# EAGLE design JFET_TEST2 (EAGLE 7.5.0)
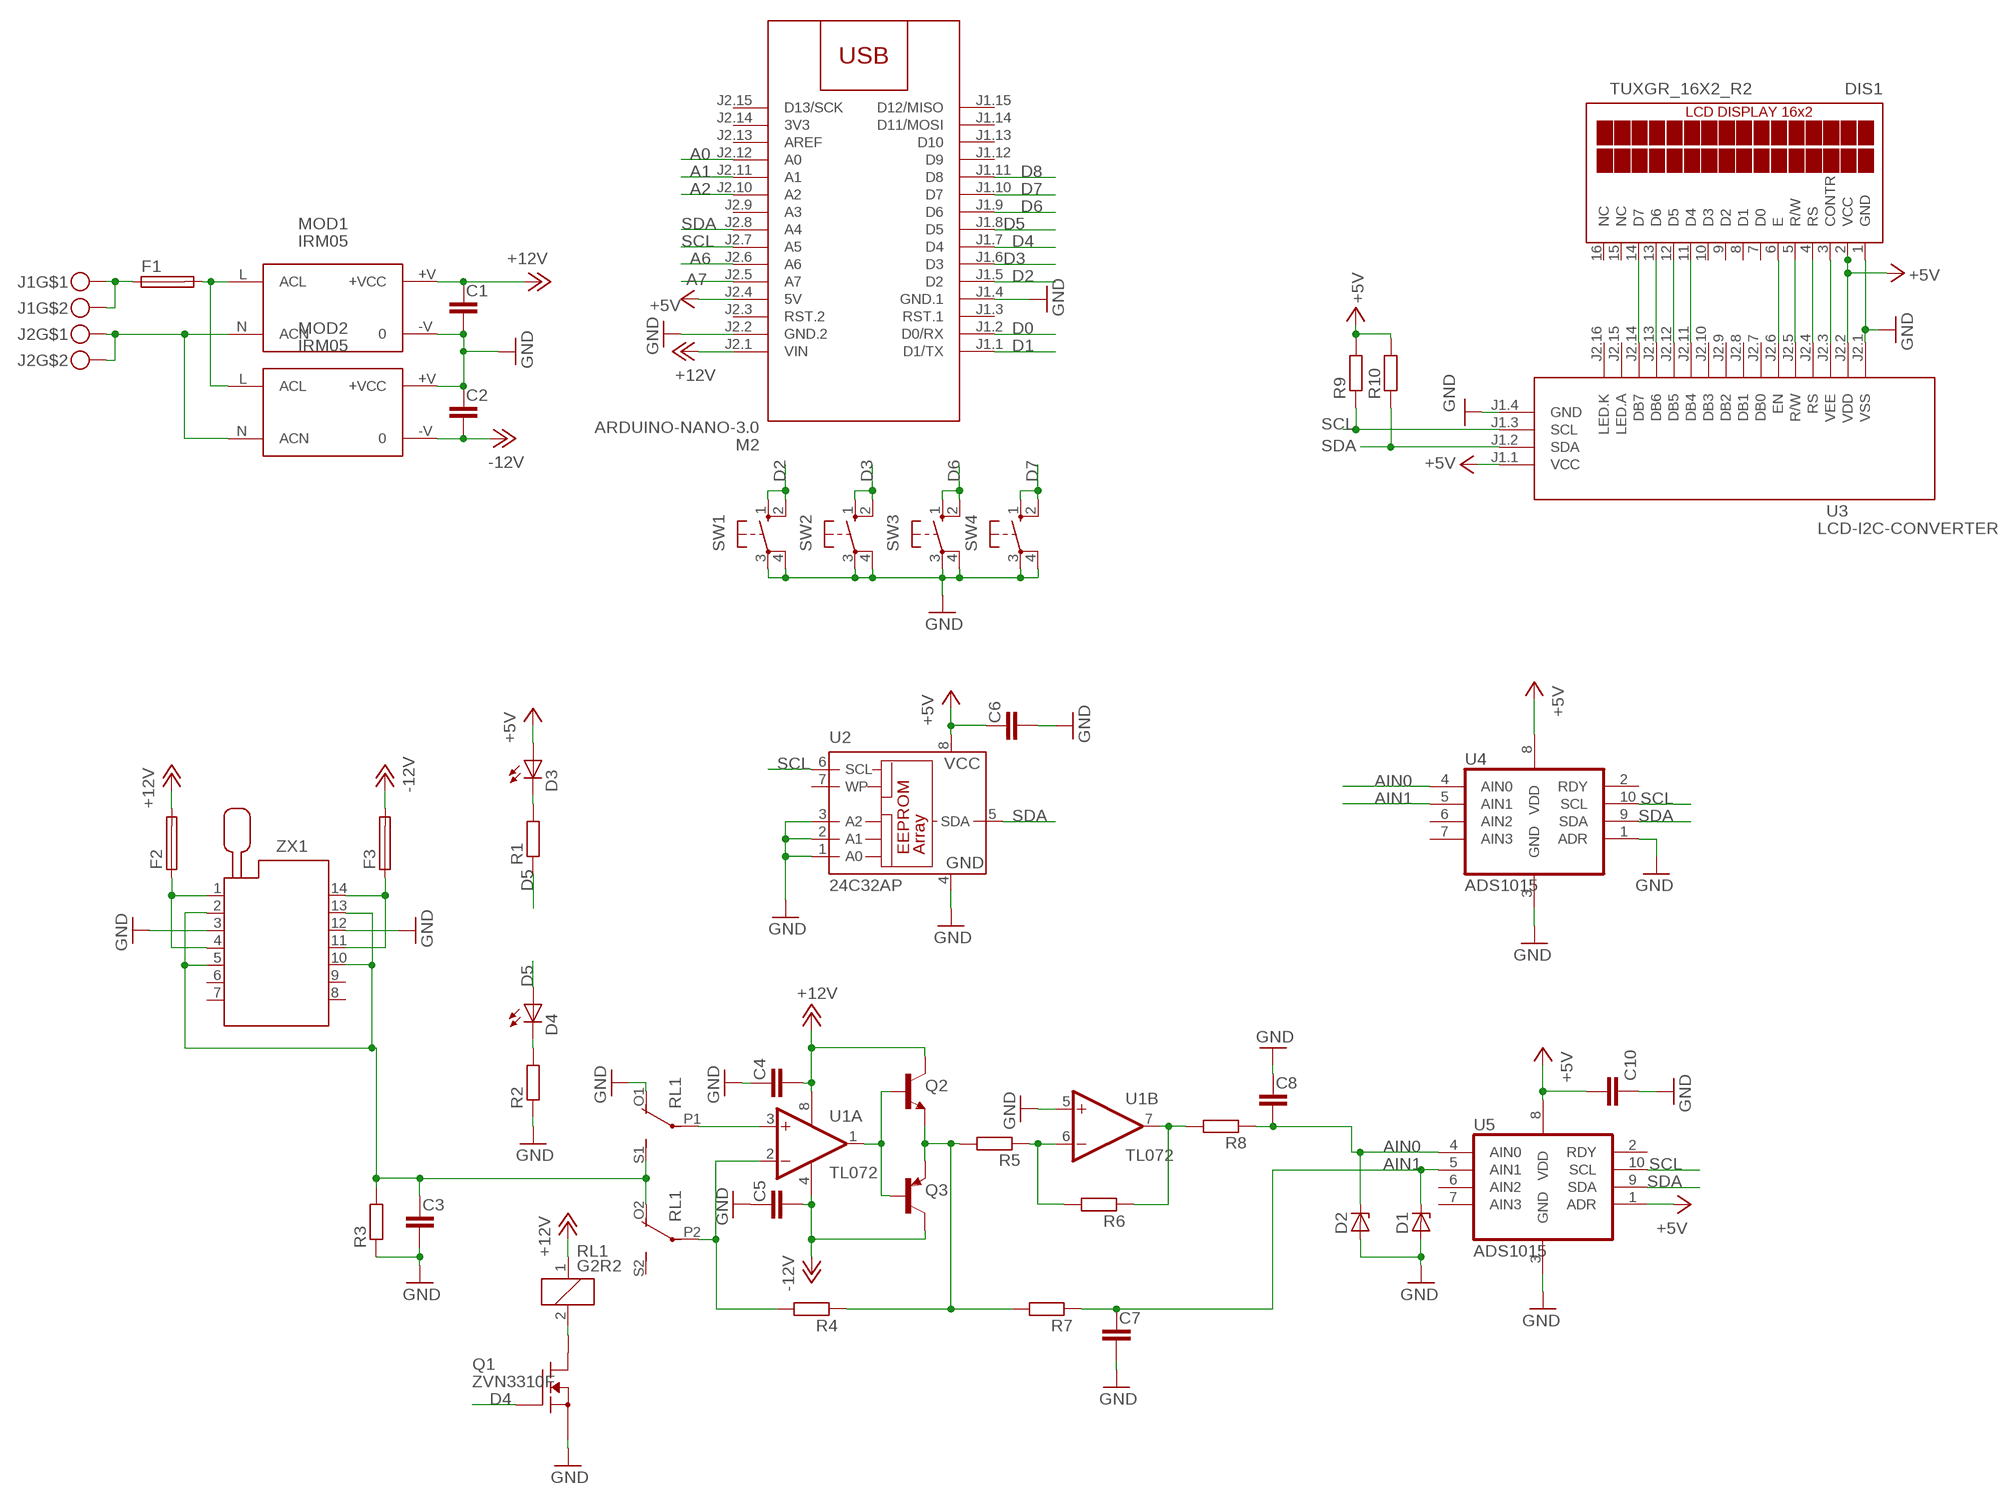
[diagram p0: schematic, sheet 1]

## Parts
C1  C-EUC1206  [C1206]
C2  C-EUC1206  [C1206]
C3  C-EUC1206  [C1206]
C4  C-EUC1206  [C1206]
C5  C-EUC1206  [C1206]
C6  C-EUC1206  [C1206]
C7  C-EUC1206  [C1206]
C8  C-EUC1206  [C1206]
C10  C-EUC1206  [C1206]
D1  BZX84CSMD  [TO236]
D2  BZX84CSMD  [TO236]
D3  LED5MM  [LED5MM]
D4  LED5MM  [LED5MM]
DIS1  TUXGR_16X2_R2  [TUXGR_16X2_R2]
F1  FUSEBLANK_5X20MM  [FUSE_HOLDER_5X20MM]
F2  FUSEBLANK_5X20MM  [FUSE_HOLDER_5X20MM]
F3  FUSEBLANK_5X20MM  [FUSE_HOLDER_5X20MM]
J1  MKDSN1,5-2-5,08  [MKDSN1,5-2-5,08]
J2  MKDSN1,5-2-5,08  [MKDSN1,5-2-5,08]
M2  ARDUINO-NANO-3.0  [ARDUINO-NANO-3.0]
MOD1  IRM05  [IRM05]
MOD2  IRM05  [IRM05]
Q1  ZVN3310F  BSS138  [SOT23]
Q2  BC817-40LT1SMD  [SOT23-BEC]
Q3  BC858ALT1SMD  [SOT23-BEC]
R1  R-EU_R1206  [R1206]
R2  R-EU_R1206  [R1206]
R3  R-EU_R1206  [R1206]
R4  R-EU_R1206  [R1206]
R5  R-EU_R1206  [R1206]
R6  R-EU_R1206  [R1206]
R7  R-EU_R1206  [R1206]
R8  R-EU_R1206  [R1206]
R9  R-EU_R1206  [R1206]
R10  R-EU_R1206  [R1206]
RL1  G2R2  [G2R2]
SW1  40-XX  [B3F-40XX]
SW2  40-XX  [B3F-40XX]
SW3  40-XX  [B3F-40XX]
SW4  40-XX  [B3F-40XX]
U1  TL072  OPA2134PA  [DIL08]
U2  24C32AP  [DIL8]
U3  LCD-I2C-CONVERTER  [LCD-I2C-CONVERTER]
U4  ADS1015  [ADS1015]
U5  ADS1015  [ADS1015]
ZX1  214-3339-00-0602J  [214-3339-00-0602J]

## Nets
+5V: C6.1 C10.2 D3.A DIS1.2(VCC) M2.J2.4(5V) R9.2 R10.2 U2.8(VCC) U3.J1.1(VCC) U3.J2.2(VDD) U4.8(VDD) U5.1(ADR) U5.8(VDD)
+12V: C1.1 C4.2 F2.2 M2.J2.1(VIN) MOD1.+V(+VCC) Q2.C RL1.1 U1.8(A:V+)
-12V: C2.2 C5.2 F3.2 MOD2.-V Q3.C U1.4(A:V-)
A0: M2.J2.12(A0)
A1: M2.J2.11(A1)
A2: M2.J2.10(A2)
A6: M2.J2.6(A6)
A7: M2.J2.5(A7)
AIN0: C8.2 D2.C R8.1 U4.4(AIN0) U5.4(AIN0)
AIN1: C7.1 D1.C R7.1 U4.5(AIN1) U5.5(AIN1)
D0: M2.J1.2(D0/RX)
D1: M2.J1.1(D1/TX)
D2: M2.J1.5(D2) SW1.1(S) SW1.2(S1)
D3: M2.J1.6(D3) SW2.1(S) SW2.2(S1)
D4: M2.J1.7(D4) Q1.3(G)
D5: D4.A M2.J1.8(D5) R1.1
D6: M2.J1.9(D6) SW3.1(S) SW3.2(S1)
D7: M2.J1.10(D7) SW4.1(S) SW4.2(S1)
D8: M2.J1.11(D8)
GND: C1.2 C2.1 C3.2 C4.1 C5.1 C6.2 C7.2 C8.1 C10.1 D1.A D2.A DIS1.1(GND) M2.J1.4(GND.1) M2.J2.2(GND.2) MOD1.-V MOD2.+V(+VCC) Q1.1(S) R2.1 R3.1 RL1.O1(2:O) SW1.3(P) SW1.4(P1) SW2.3(P) SW2.4(P1) SW3.3(P) SW3.4(P1) SW4.3(P) SW4.4(P1) U1.5(B:+IN) U2.1(A0) U2.2(A1) U2.3(A2) U2.4(GND) U3.J1.4(GND) U3.J2.1(VSS) U4.1(ADR) U4.3(GND) U5.3(GND) ZX1.3 ZX1.12
N$1: DIS1.14(D7) U3.J2.14(DB7)
N$2: DIS1.13(D6) U3.J2.13(DB6)
N$3: DIS1.12(D5) U3.J2.12(DB5)
N$4: DIS1.11(D4) U3.J2.11(DB4)
N$5: DIS1.6(E) U3.J2.6(EN)
N$6: DIS1.5(R/W) U3.J2.5(R/W)
N$7: DIS1.4(RS) U3.J2.4(RS)
N$10: DIS1.3(CONTR) U3.J2.3(VEE)
N$11: C3.1 R3.2 RL1.O2(3:O) RL1.S1(2:S) ZX1.2 ZX1.5 ZX1.10 ZX1.13
N$13: D4.K(C) R2.2
N$14: D3.K(C) R1.2
N$15: Q1.2(D) RL1.2
N$16: RL1.P1(2:P) U1.3(A:+IN)
N$17: R4.2 RL1.P2(3:P) U1.2(A:-IN)
N$18: Q2.B Q3.B U1.1(A:OUT)
N$19: Q2.E Q3.E R4.1 R5.2 R7.2
N$20: F1.1 J1.1 J1.2
N$21: F1.2 MOD1.L(ACL) MOD2.L(ACL)
N$24: R5.1 R6.2 U1.6(B:-IN)
N$25: R6.1 R8.2 U1.7(B:OUT)
N$26: J2.1 J2.2 MOD1.N(ACN) MOD2.N(ACN)
N$27: F2.1 ZX1.1 ZX1.4
N$28: F3.1 ZX1.11 ZX1.14
SCL: M2.J2.7(A5) R9.1 U2.6(SCL) U3.J1.3(SCL) U4.10(SCL) U5.10(SCL)
SDA: M2.J2.8(A4) R10.1 U2.5(SDA) U3.J1.2(SDA) U4.9(SDA) U5.9(SDA)
Unconnected: DIS1.7(D0) DIS1.8(D1) DIS1.9(D2) DIS1.10(D3) DIS1.15(NC) DIS1.16(NC) M2.J1.3(RST.1) M2.J1.12(D9) M2.J1.13(D10) M2.J1.14(D11/MOSI) M2.J1.15(D12/MISO) M2.J2.3(RST.2) M2.J2.9(A3) M2.J2.13(AREF) M2.J2.15(D13/SCK) RL1.S2(3:S) U2.7(WP) U3.J2.7(DB0) U3.J2.8(DB1) U3.J2.9(DB2) U3.J2.10(DB3) U3.J2.15(LED.A) U3.J2.16(LED.K) U4.2(RDY) U4.6(AIN2) U4.7(AIN3) U5.2(RDY) U5.6(AIN2) U5.7(AIN3) ZX1.6 ZX1.7 ZX1.8 ZX1.9

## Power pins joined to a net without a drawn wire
3V3: M2.J2.14(3V3)

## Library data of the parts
C1-C8 C10 = rcl:C-EU: CAPACITOR, European symbol
D1 D2 = diode:BZX84CSMD: Z DIODE
D3 D4 = led:LED: LED
DIS1 = display-lcd:TUXGR_16X2_R2: Tuxgraphics LCD display 16x2 characters reflective, without background light Source: tuxgr_12x2_r2.pdf; OC_FARNELL: unknown; OC_NEWARK: unknown
F1-F3 = fuse:FUSE: Fuse; OC_FARNELL: unknown; OC_NEWARK: unknown
J1 J2 = con-phoenix-508:MKDSN1,5-2-5,08
M2 = diy-modules:ARDUINO-NANO-3.0: Arduino Nano 3.0 and compatible devices More details available here: https://www.arduino.cc/en/Main/ArduinoBoardNano Click here to find device on ebay.com
MOD1 MOD2 = acdc:IRM05: ACDC connector
Q1 = transistor-fet:BSS138
Q2 = transistor-npn:BC817*: NPN Transistor
Q3 = transistor-pnp:BC858*: PNP Transistror
R1-R10 = rcl:R-EU_: RESISTOR, European symbol
RL1 = relay:G2R2: RELAY 2 x switch, Omron; MF: OMRON COMPONENTS USA; MPN: G2R-2-DC6; OC_FARNELL: unknown; OC_NEWARK: 89C5317
SW1-SW4 = switch-omron:40-XX: OMRON SWITCH; MF: OMRON COMPONENTS USA; MPN: B3F-4000; OC_FARNELL: 176434; OC_NEWARK: 36K3105
U1 = linear:OPA2*: Dual Operational Amplifier Low Power, Single-Supply, Rail-To-Rail Operational Amplifier Source: http://focus.ti.com/lit/ds/symlink/opa2345.pdf http://focus.ti.com .. opa241.pdf http://focus.ti.com/lit/ds/symlink/opa2134.pdf
U2 = microchip:24*: Serial EEPROM I2C; MPN: AT24C32C-PU; OC_FARNELL: 1362652; OC_NEWARK: 50M3325
U3 = diy-modules:LCD-I2C-CONVERTER: I2C Bus to 4-Bit Parallel LCD Interface with LED backlight driver
U4 U5 = burr-brown:ADS1015: 12BIT I2C DAC
ZX1 = con-3m:214-3339-00-0602J: Zero Insertion Force Socked Source: http://www.3M.com/ehpd; MF: 3M; MPN: 214-3339-00-0602J; OC_FARNELL: 1247151; OC_NEWARK: 85K7793

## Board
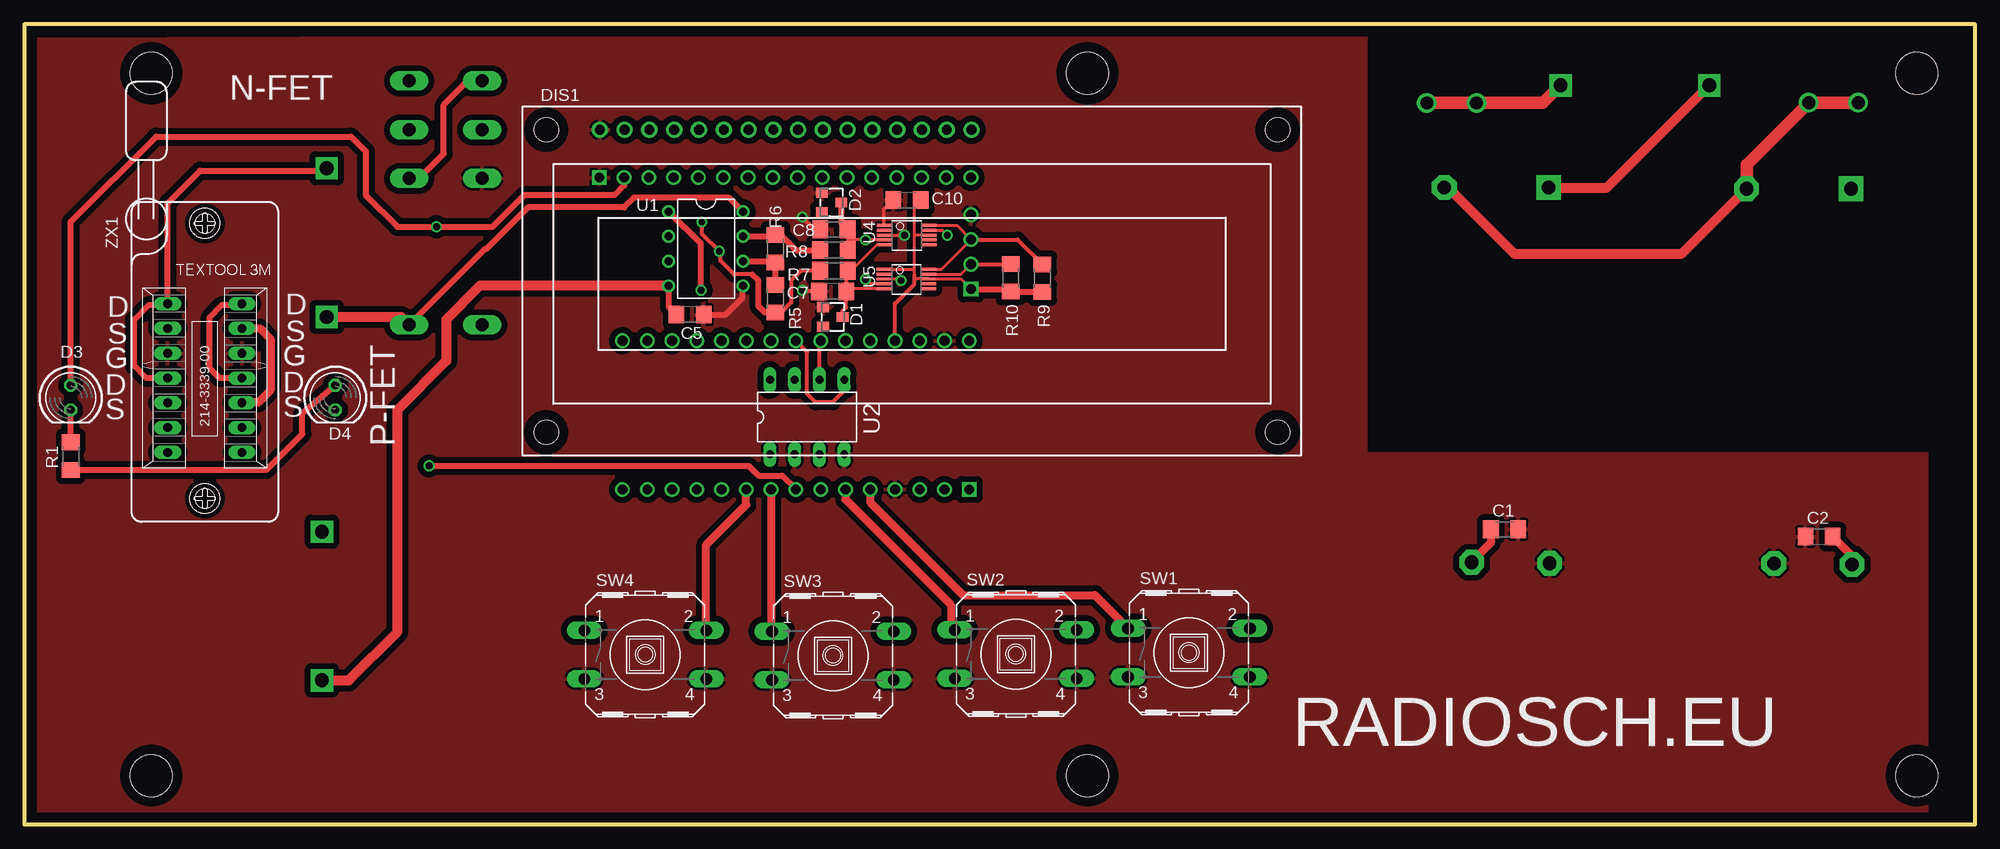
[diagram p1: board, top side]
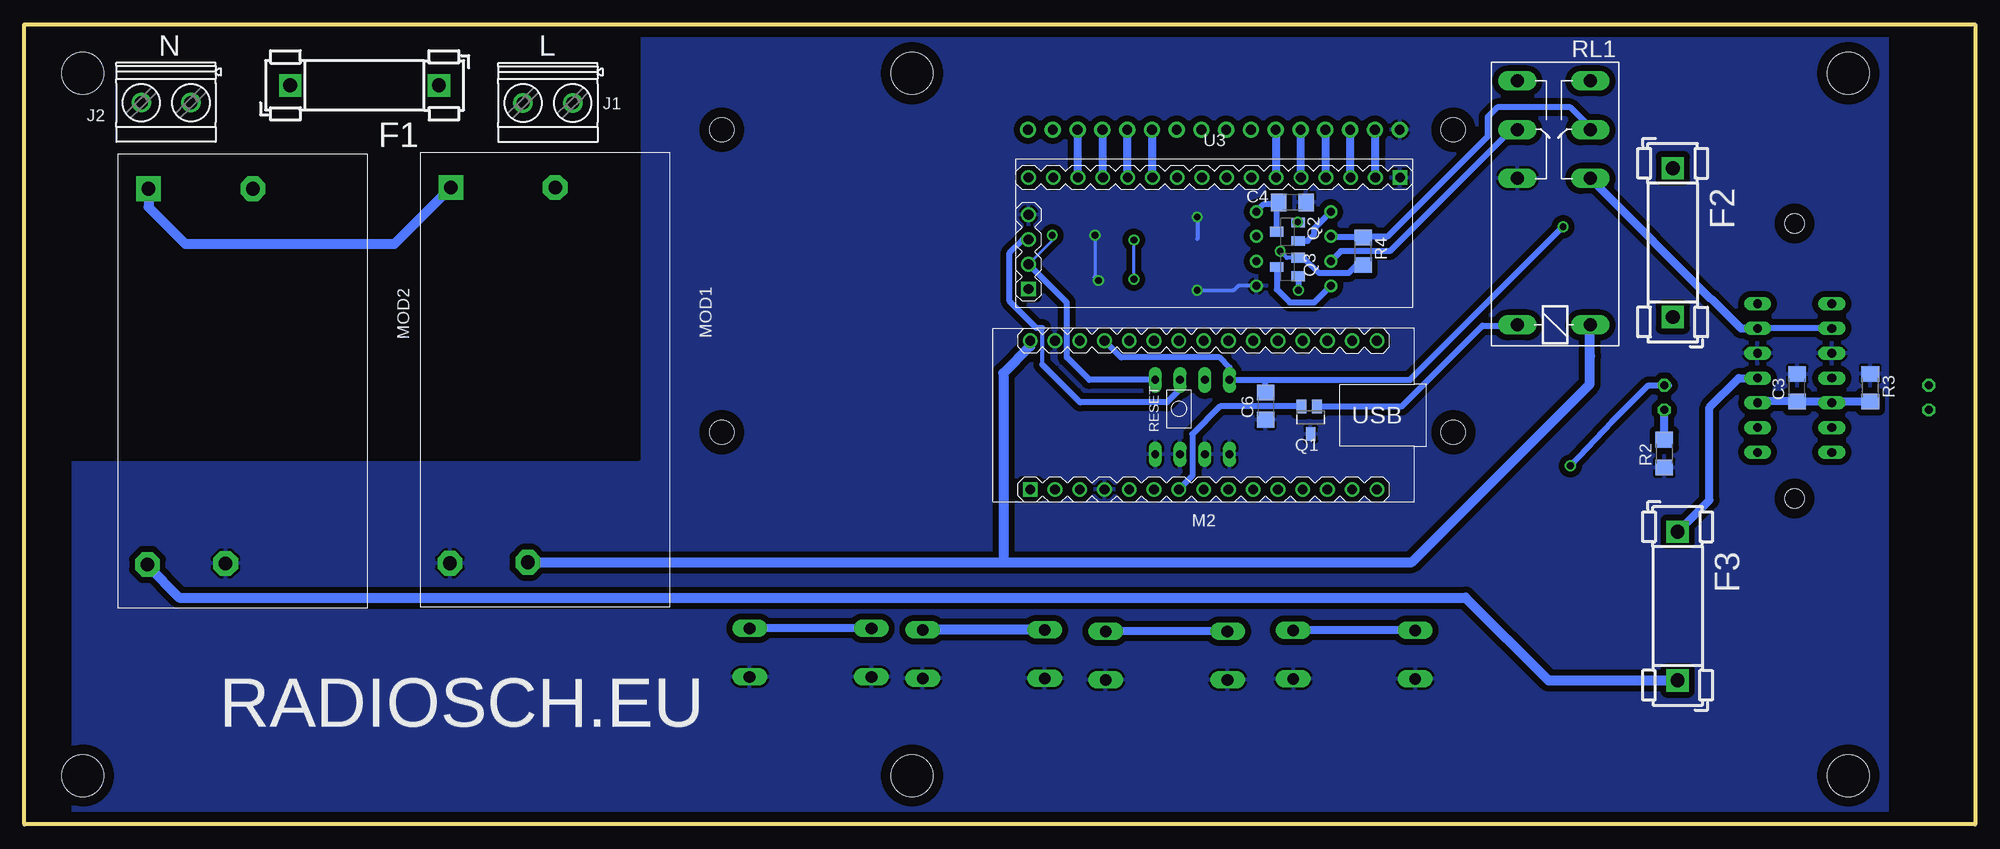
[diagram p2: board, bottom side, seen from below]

Size 200 x 82 mm. Coordinates in mm from the lower left corner, seen from the top.
Outline: 0,0 200,0 200,82 0,82 0,0
Copper layers (1*16): Top 0.035mm / dielectric 1.5mm / Bottom 0.035mm
Design rules "default *": minimum track width 10mil, minimum drill 24mil, track to track 4mil, track to pad 6mil, pad to pad 4mil, via to via 8mil, smd to smd 8mil, copper to edge 40mil, drill to drill 8mil, minimum pad ring 10mil, minimum via ring 8mil, stop-mask expansion 4mil, vias tented up to drill 0mil, thermal gap 10mil
Holes 4.3 mm at 13,77 13,5 109,5 194,5 109,77 194,77

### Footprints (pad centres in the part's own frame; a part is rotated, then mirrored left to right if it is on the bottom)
C1206 = smd 1.6 x 1.8: 1 -1.4,0; 2 1.4,0
TO236 = smd 1 x 1.2: A -1,-1; C 0,1; NC 1,-1
LED5MM = drill 0.813 octagon: A -1.27,0; K 1.27,0
TUXGR_16X2_R2 = drill 1 pad 1.676: 1 -32,15.5; 2 -29.46,15.5; 3 -26.92,15.5; 4 -24.38,15.5; 5 -21.84,15.5; 6 -19.3,15.5; 7 -16.76,15.5; 8 -14.22,15.5; 9 -11.68,15.5; 10 -9.14,15.5; 11 -6.6,15.5; 12 -4.06,15.5; 13 -1.52,15.5; 14 1.02,15.5; 15 3.56,15.5; 16 6.1,15.5 | hole 2.5: -37.5,-15.5; 37.5,-15.5; -37.5,15.5; 37.5,15.5
FUSE_HOLDER_5X20MM = drill 1.422 pad 2.286 square: 1 0,0; 2 15.24,0
MKDSN1,5-2-5,08 = drill 1.3 pad 2: 1 -2.561,0.025; 2 2.519,0.025
ARDUINO-NANO-3.0 = drill 1 square: J1.1 17.78,7.62 | drill 1: J1.2 15.24,7.62; J1.3 12.7,7.62; J1.4 10.16,7.62; J1.5 7.62,7.62; J1.6 5.08,7.62; J1.7 2.54,7.62; J1.8 0,7.62; J1.9 -2.54,7.62; J1.10 -5.08,7.62; J1.11 -7.62,7.62; J1.12 -10.16,7.62; J1.13 -12.7,7.62; J1.14 -15.24,7.62; J1.15 -17.78,7.62; J2.1 17.78,-7.62; J2.2 15.24,-7.62; J2.3 12.7,-7.62; J2.4 10.16,-7.62; J2.5 7.62,-7.62; J2.6 5.08,-7.62; J2.7 2.54,-7.62; J2.8 0,-7.62; J2.9 -2.54,-7.62; J2.10 -5.08,-7.62; J2.11 -7.62,-7.62; J2.12 -10.16,-7.62; J2.13 -12.7,-7.62; J2.14 -15.24,-7.62; J2.15 -17.78,-7.62
IRM05 = drill 1.4 pad 2.54 octagon: +V 42,-14.5; -V 42.1,-22.5; N 3.6,-11.7 | drill 1.4 pad 2.54 square: L 3.6,-22.4
SOT23 = smd 1 x 1.4: 1 0,1.735; 2 -0.632,-1.1; 3 0.95,-1.1
SOT23-BEC = smd 1 x 1.4: B -0.95,-1.1; C 0,1.1; E 0.95,-1.1
R1206 = smd 1.6 x 1.803: 1 -1.422,0; 2 1.422,0
G2R2 = drill 1.321 long: 1 -2.54,-3.683; 2 -2.54,3.81; O1 12.471,3.81; O2 12.471,-3.683; P1 17.45,3.81; P2 17.45,-3.683; S1 22.454,3.81; S2 22.454,-3.683
B3F-40XX = drill 1.194 long: 1 -6.248,2.489; 2 6.248,2.489; 3 -6.248,-2.489; 4 6.248,-2.489
DIL08 = drill 0.813 pad 1.27: 1 -3.81,-3.81; 2 -1.27,-3.81; 3 1.27,-3.81; 4 3.81,-3.81; 5 3.81,3.81; 6 1.27,3.81; 7 -1.27,3.81; 8 -3.81,3.81
DIL8 = drill 0.813 long: 1 -3.81,-3.81; 2 -1.27,-3.81; 3 1.27,-3.81; 4 3.81,-3.81; 5 3.81,3.81; 6 1.27,3.81; 7 -1.27,3.81; 8 -3.81,3.81
LCD-I2C-CONVERTER = drill 1 square: J1.1 -19.05,-5.08; J2.1 19.05,6.35 | drill 1: J1.2 -19.05,-2.54; J1.3 -19.05,0; J1.4 -19.05,2.54; J2.2 16.51,6.35; J2.3 13.97,6.35; J2.4 11.43,6.35; J2.5 8.89,6.35; J2.6 6.35,6.35; J2.7 3.81,6.35; J2.8 1.27,6.35; J2.9 -1.27,6.35; J2.10 -3.81,6.35; J2.11 -6.35,6.35; J2.12 -8.89,6.35; J2.13 -11.43,6.35; J2.14 -13.97,6.35; J2.15 -16.51,6.35; J2.16 -19.05,6.35
ADS1015 = smd 0.3 x 1.5: 1 -1.905,-2.616; 2 -1.405,-2.616; 3 -0.905,-2.616; 4 -0.405,-2.616; 5 0.095,-2.616; 6 0.095,1.984; 7 -0.405,1.984; 8 -0.905,1.984; 9 -1.405,1.984; 10 -1.905,1.984
214-3339-00-0602J = drill 0.9 long: 1 -7.62,-3.81; 2 -5.08,-3.81; 3 -2.54,-3.81; 4 0,-3.81; 5 2.54,-3.81; 6 5.08,-3.81; 7 7.62,-3.81; 8 7.62,3.81; 9 5.08,3.81; 10 2.54,3.81; 11 0,3.81; 12 -2.54,3.81; 13 -5.08,3.81; 14 -7.62,3.81 | hole 2: 12.35,0; -15.85,0

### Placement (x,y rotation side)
C1  151.75,30.25 0 top
C2  184,29.5 0 top
C3  18.25,44.75 90 bottom
C4  70,63.75 180 bottom
C5  68.25,52.25 180 top
C6  72.75,42.88 270 bottom
C7  82.88,54.62 180 top
C8  83,61 0 top
C10  90.5,64 0 top
D1  82.88,52 270 top
D2  82.75,63.75 270 top
D3  4.75,43.75 270 top
D4  31.88,43.75 270 top
DIS1  91,55.7 0 top
F1  157.5,75.75 180 bottom
F2  31,67.25 270 bottom
F3  30.5,30 270 bottom
J1  146.35,73.97 180 bottom
J2  185.5,74 180 bottom
M2  79.1,41.95 180 bottom
MOD1  133.88,68.88 270 bottom
MOD2  164.88,68.75 270 bottom
Q1  68.12,41.75 180 bottom
Q2  70.5,60.75 90 bottom
Q3  70.5,57.12 90 bottom
R1  4.75,37.75 90 top
R2  31.88,38 90 bottom
R3  10.75,44.75 270 bottom
R4  62.75,58.75 90 bottom
R5  77,53.88 270 top
R6  77,59 270 top
R7  83,56.75 180 top
R8  83,58.88 180 top
R9  104.38,55.97 270 top
R10  101.12,56.03 270 top
RL1  43.12,53.75 90 bottom
SW1  119.4,17.6 0 top
SW2  101.65,17.45 0 top
SW3  82.9,17.3 0 top
SW4  63.65,17.4 0 top
U1  69.88,59 270 top
U2  80.25,41.75 0 top
U3  78,59.95 0 bottom
U4  90.78,59.5 270 top
U5  90.75,55 270 top
ZX1  18.5,45.75 270 top

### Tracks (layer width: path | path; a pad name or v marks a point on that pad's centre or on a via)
+5V  (via drill 0.7)
  Top 0.305: U5.1 91.22,56.91 91.25,56.88 | 91.25,56.88 91.25,60.5 | 91.25,60.5 91.25,63.35 C10.2 | U4.8 91.34,60.41 91.25,60.5 | 91.25,56.88 91.25,56.25 91.25,56.12 91.47,55.91 U5.8 96.02,55.91 U3.J1.1
  Top 0.406: M2.J2.4 89.26,53.39 91.25,55.38 91.25,56.25
  Top 0.61: U3.J1.1 100.86,54.87 R10.2 104.33,54.6 R9.2 | U3.J2.2 61.49,65.49 60.5,64.5 51.25,64.5 48,61.25 v42.25,61.25 38.25,61.25 35,64.5 35,69 33.5,70.5 13.5,70.5 4.75,61.75 D3.A
  Bottom 0.61: M2.J2.4 87.56,47.88 77.5,47.88 76.44,46.81 U2.8 72.88,45.56 | 72.88,45.56 57.94,45.56 v42.25,61.25 | C6.1 72.75,45.44 72.88,45.56
  Bottom 0.813: U3.J2.2 61.49,71.15 DIS1.2
+12V
  Top 0.61: RL1.1 47.23,59 47.38,59 51.62,63.25 61.5,63.25 62.5,64.25 72.25,64.25 U1.8
  Top 0.813: C1.1 150.35,28.85 MOD1.+V
  Top 1.016: F2.2 38.64,52.01 RL1.1
  Bottom 0.61: Q2.C 71.6,63.55 | 71.6,63.55 C4.2 | 71.6,63.55 72.94,63.55 U1.8
  Bottom 1.016: MOD1.+V 99.62,26.88 | 99.62,26.88 57.75,26.88 39.5,45.12 39.5,48 | 39.5,48 39.5,51.15 RL1.1 | 39.49,48.01 39.5,48 | M2.J2.1 96.88,49 99.62,46.25 99.62,26.88
-12V
  Top 0.61: U1.4 66.06,53.03 C5.2
  Top 0.813: MOD2.-V 187.38,27.52 C2.2
  Top 1.016: U1.4 66,55.25 46.75,55.25 43.25,51.75 43.25,47.5 38.25,42.5 38.25,19.75 33.26,14.76 F3.2
  Bottom 0.61: Q3.C 71.6,54.85 70.25,53.5 67.75,53.5 U1.4
  Bottom 1.016: MOD2.-V 187.38,26.5 184.12,23.25 52.25,23.25 43.75,14.75 F3.2
AIN0  (via drill 0.7)
  Top 0.305: R8.1 84.42,59.75 | 84.42,59.75 84.42,60.98 C8.2 | U4.4 v86.25,59.91 84.58,59.91 84.42,59.75 | U5.4 86.72,55.41 v86.25,55.88
  Top 0.61: D2.C 83.75,61.65 C8.2
  Bottom 0.305: v86.25,55.88 v86.25,59.91
AIN1
  Top 0.305: U5.5 84.56,54.91 C7.1 | U4.5 87.41,59.41 85,57 84.67,57 R7.1
  Top 0.406: D1.C 83.88,52.62 84.25,53 84.25,54.6 C7.1 84.28,56.6 R7.1
D2
  Top 0.813: M2.J1.5 86.72,33.03 96.25,23.5 109.74,23.5 SW1.1
  Bottom 0.813: SW1.1 SW1.2
D3
  Top 0.813: M2.J1.6 84.18,33.32 95,22.5 95,20.34 SW2.1
  Bottom 1.016: SW2.1 SW2.2
D4
  Bottom 0.61: Q1.3 77.4,42.85 80.25,40 80.25,35.72 M2.J1.7
D5  (via drill 0.7)
  Top 0.61: v41.5,36.75 74.25,36.75 75.25,35.75 77.68,35.75 M2.J1.8 | D4.A 28.5,42.15 28.5,40 24.83,36.33 R1.1
  Bottom 0.61: v41.5,36.75 37.25,41.25 33.5,45 31.39,45 D4.A
D6
  Top 0.813: M2.J1.9 76.56,19.88 SW3.1
  Bottom 0.813: SW3.1 SW3.2
D7
  Top 0.813: SW4.2 69.9,28.65 74,32.75 74,34.31 M2.J1.10
  Bottom 0.813: SW4.1 SW4.2
GND  (via drill 0.7)
  Top 0.305: U5.3 90.03,55.91 v89.88,55.75 | U4.3 90.22,60.41 v90.25,60.38 | U4.1 88.16,62.09 88.12,62.12 88.12,63.12
  Top 0.406: 88.16,63.06 C10.1 | C7.2 79.88,54.62 v79.75,54.75 | C8.1 81,61 v79.75,62.25
  Top 0.61: C5.1 71.88,52.25 73.62,54 73.62,55.13 U1.5
  Bottom 0.305: 90.38,56.12 90,55.75 v89.88,55.75 90.25,56.12 v90.25,60.38
  Bottom 0.406: v79.75,54.75 76,54.75 75.5,55.25 73.75,55.25 U1.5 | v79.75,62.25 79.75,60
  pour Bottom (isolate 0.61): 9,81 195,81 195,1.5 9,1.5
  cutout Bottom: 137,81.5 195,81.5 195.5,37.5 137,37.5
  pour Top (isolate 0.61): 1,80.5 137.5,81 137.5,38 195,38 195,1 1,0.5
N$1
  Bottom 0.813: U3.J2.14 91.97,71.15 DIS1.14
N$2
  Bottom 0.813: U3.J2.13 89.43,71.15 DIS1.13
N$3
  Bottom 0.813: U3.J2.12 86.89,71.15 DIS1.12
N$4
  Bottom 0.813: U3.J2.11 84.35,71.15 DIS1.11
N$5
  Bottom 0.813: U3.J2.6 71.65,71.15 DIS1.6
N$6
  Bottom 0.813: U3.J2.5 69.11,71.15 DIS1.5
N$7
  Bottom 0.813: U3.J2.4 66.57,71.15 DIS1.4
N$10
  Bottom 0.813: U3.J2.3 64.03,71.15 DIS1.3
N$11
  Top 0.61: RL1.O2 40.47,66.22 43,68.75 43,73.75 45.25,76 46.73,76 RL1.S1
  Top 0.813: ZX1.13 24.17,50.83 25.25,49.75 25.25,44.5 24,43.25 22.35,43.25 ZX1.10
  Bottom 0.61: ZX1.2 ZX1.13
  Bottom 0.813: R3.2 14.57,43.33 ZX1.5 14.83,43.35 C3.1 22.17,43.35 ZX1.10 | ZX1.13 24,50.83 27,53.83 27.08,53.83 38.75,65.5 38.75,65.53 RL1.O2
N$13
  Bottom 0.813: R2.2 D4.K
N$14
  Top 0.61: R1.2 D3.K
N$15
  Bottom 0.61: Q1.2 58.77,42.85 50.5,51.12 47.02,51.12 RL1.2
N$16
  Bottom 0.61: RL1.P1 47.55,71.2 60,58.75 65.05,58.75 U1.3
N$17
  Bottom 0.61: RL1.P2 39.44,71.44 41.5,73.5 49,73.5 50,72.5 50,70.5 60.25,60.25 62.67,60.25 R4.2 65.97,60.17 U1.2
N$18  (via drill 0.7)
  Top 0.61: v69.38,54.75 69.38,59.5 U1.1
  Bottom 0.61: Q2.B 68.45,59.8 67.75,60.5 67.75,61.12 U1.1 | Q3.B 69.4,54.78 v69.38,54.75
N$19  (via drill 0.7)
  Top 0.406: v69.45,61.75 69.45,60.55 v71.25,58.75 71.38,58.62 71.38,57.75 72.75,56.38 74.62,56.38 | R7.2 79.62,56.75 78.62,55.75 78.62,53.5 77.62,52.5 77.05,52.5 R5.2
  Top 0.61: R5.2 75.92,52.45 75.25,53.12 75.25,55.75 74.62,56.38
  Bottom 0.406: Q3.E 70.58,58.08 v71.25,58.75 | 69.25,61.75 v69.45,61.75 Q2.E
  Bottom 0.61: R4.1 63.42,57.33 64.25,56.5 67.25,56.5 68.75,58 69.33,58 Q3.E
N$20
  Top 1.27: J1.1 J1.2 155.7,73.95 F1.1
N$21
  Top 1.016: MOD1.L 162.26,65.28 F1.2
  Bottom 1.016: MOD2.L 187.28,63.28 183.5,59.5 162.05,59.5 MOD1.L
N$24
  Top 0.61: R5.1 R6.2 76.1,57.73 U1.6
N$25
  Top 0.61: U1.7 76.35,60.27 R6.1 77.7,60.3 79.12,58.88 R8.2
N$26
  Top 1.016: MOD1.N 145.97,65.28 152.75,58.5 169.93,58.5 MOD2.N
  Top 1.27: MOD2.N 176.57,67.61 J2.1 J2.2
N$27
  Top 0.61: ZX1.4 12.5,45.75 11.25,47 11.25,51.75 12.75,53.25 14.57,53.25 ZX1.1 14.69,63.69 18,67 30.75,67 F2.1
N$28
  Top 0.61: ZX1.11 20,45.75 19,46.75 19,52 20.25,53.25 22.19,53.25 ZX1.14
  Bottom 0.813: F3.1 27.25,33.25 27.25,42.75 24.25,45.75 ZX1.11
SCL
  Top 0.305: U4.10 95.59,61.41 U3.J1.3 94,56.91 U5.10
  Top 0.406: U3.J1.3 101.82,59.95 R9.1 | U2.6 81.52,49.45 M2.J2.7
  Bottom 0.406: 95.62,47.12 95.62,50.88
  Bottom 0.61: U2.6 81.52,44.61 82.88,43.25 91.75,43.25 95.62,47.12 | 95.62,50.88 96.25,50.88 99,53.62 99,58.58 97.62,59.95 U3.J1.3
SDA  (via drill 0.7)
  Top 0.305: U5.9 96.05,56.41 U3.J1.2 | U4.9 94.09,60.91 v94.62,60.38
  Top 0.406: U3.J1.2 101.09,57.41 R10.1 | U2.5 84.06,44.44 82.88,43.25 81.12,43.25 80.25,44.12 80.25,48.42 M2.J2.8
  Bottom 0.305: v94.62,60.38 94.62,59.83 U3.J1.2
  Bottom 0.61: U2.5 90.81,45.56 93.12,47.88 93.12,53.48 U3.J1.2

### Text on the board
tPlace: N-FET | OUT1 | D | D | S | S | G | G | D | D | S | S | P-FET | RADIOSCH.EU
bPlace: L | N | RADIOSCH.EU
